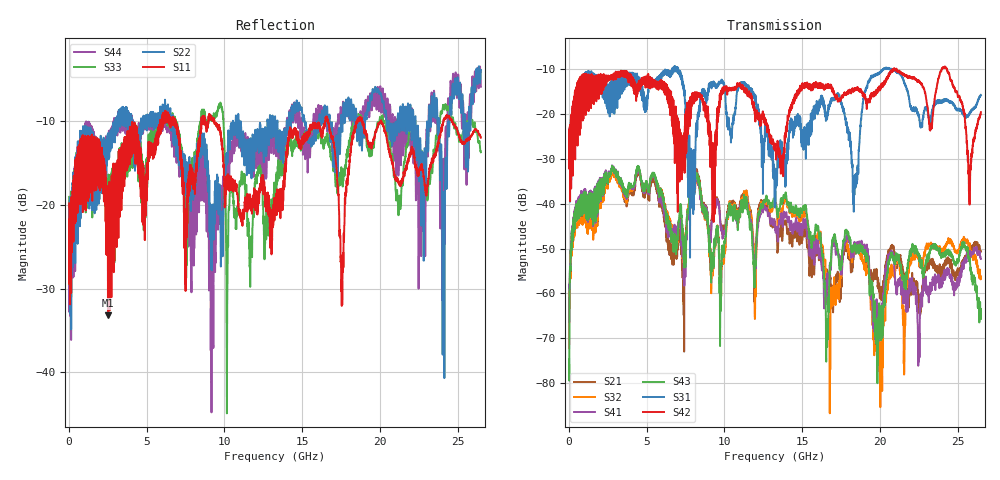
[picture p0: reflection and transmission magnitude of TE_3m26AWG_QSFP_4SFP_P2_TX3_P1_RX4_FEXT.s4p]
!Agilent Technologies,N5222A,MY51421691,A.10.00.00
!Agilent N5222A: A.10.00.00
!Date: Friday, January 30, 2015 12:37:18
!Correction: S11(Full 4 Port(1,2,3,4))
!S12(Full 4 Port(1,2,3,4))
!S13(Full 4 Port(1,2,3,4))
!S14(Full 4 Port(1,2,3,4))
!S21(Full 4 Port(1,2,3,4))
!S22(Full 4 Port(1,2,3,4))
!S23(Full 4 Port(1,2,3,4))
!S24(Full 4 Port(1,2,3,4))
!S31(Full 4 Port(1,2,3,4))
!S32(Full 4 Port(1,2,3,4))
!S33(Full 4 Port(1,2,3,4))
!S34(Full 4 Port(1,2,3,4))
!S41(Full 4 Port(1,2,3,4))
!S42(Full 4 Port(1,2,3,4))
!S43(Full 4 Port(1,2,3,4))
!S44(Full 4 Port(1,2,3,4))
!S4P File: Measurements: <S11,S12,S13,S14>,
!<S21,S22,S23,S24>,
!<S31,S32,S33,S34>,
!<S41,S42,S43,S44>:
# Hz S  dB  R 50.0
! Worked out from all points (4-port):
!   2650 points, 10 MHz to 26.5 GHz, reference 50 ohm
!   strongest paths, dB at 10 MHz, 6.63 GHz, 13.26 GHz, 19.88 GHz, 26.5 GHz:
!     S42: -25.1, -19.3, -27.0, -14.8, -19.5
!     S31: -24.9, -10.4, -34.2, -10.8, -15.7
!     S43: -74.8, -46.7, -40.6, -69.3, -65.7
!     S41: -66.5, -46.8, -45.4, -69.2, -52.3
!     S32: -72.2, -45.2, -40.4, -72.2, -56.7
!     S21: -64.7, -50.8, -45.1, -58.9, -50.6
!   lowest |S11| = -33.2 dB at 2.51 GHz (marker M1), VSWR 1.04, Z = 51.1 - j1.94 ohm
!   |S11| at or under -10 dB: start of sweep to 5.869 GHz; 9.356 GHz to 16.5 GHz (7.14 GHz wide, 55.2 % of centre); 20.09 GHz to 24.09 GHz (4 GHz wide, 18.1 % of centre)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
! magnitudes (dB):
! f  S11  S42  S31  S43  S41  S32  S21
! 10 MHz  -19.8  -25.1  -24.9  -74.8  -66.5  -72.2  -64.7
! 2.51 GHz  -33.2  -12.6  -19.7  -34.7  -34.3  -35.1  -34.7
! 15.15 GHz  -11.8  -14.2  -22.9  -41.1  -45.4  -42.4  -47.0
! 16.61 GHz  -9.9  -13.6  -20.9  -71.9  -56.2  -58.7  -55.1
! 18.39 GHz  -10.6  -14.3  -33.6  -48.9  -48.8  -49.3  -50.2
! 20.03 GHz  -10.2  -14.5  -10.6  -69.9  -70.0  -85.4  -60.4
! 26.5 GHz  -12.0  -19.5  -15.7  -65.7  -52.3  -56.7  -50.6
